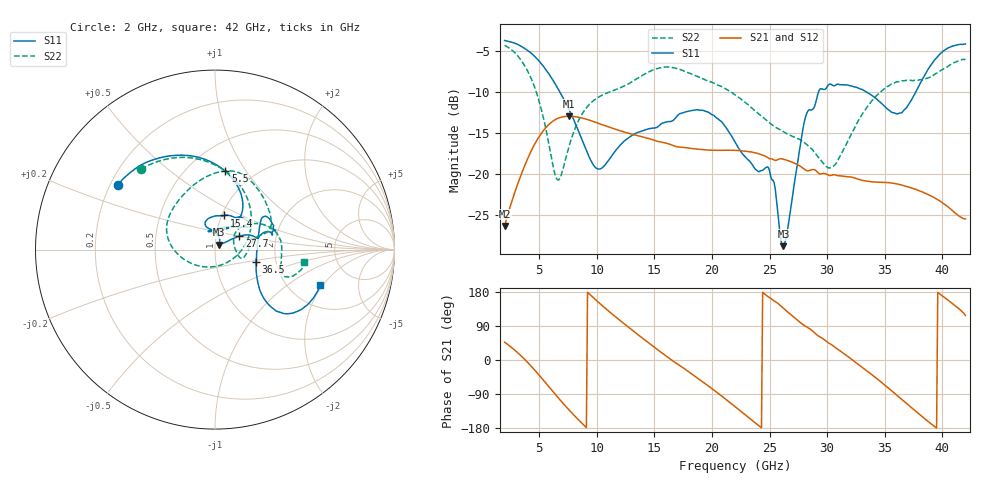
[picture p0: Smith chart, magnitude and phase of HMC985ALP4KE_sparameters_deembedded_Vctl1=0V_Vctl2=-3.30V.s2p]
!s2p File: Measurements: S11, S21, S12, S22
# GHz S dB R 50.0
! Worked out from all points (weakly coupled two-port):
!   401 points, 2 GHz to 42 GHz, reference 50 ohm
!   highest |S21| = -12.95 dB at 7.6 GHz (marker M1); lowest = -26.3 dB at 2 GHz (marker M2)
!   lowest |S11| = -28.8 dB at 26.2 GHz (marker M3), VSWR 1.08, Z = 52.3 + j2.96 ohm
!   |S11| at or under -10 dB: 6.795 GHz to 29.25 GHz (22.46 GHz wide, 125 % of centre); 33.41 GHz to 37.69 GHz (4.286 GHz wide, 12.1 % of centre)
!   |S22| runs from -20.7 to -4.3 dB; largest |S21 - S12| = 0.00059
!   S11 on the Smith chart (normalised r, x): 2 GHz: 0.23, +0.29; 5.5 GHz: 0.75, +0.81; 15.4 GHz: 1.03, +0.41; 27.7 GHz: 1.30, +0.20; 36.5 GHz: 1.57, -0.23; 42 GHz: 2.93, -1.89
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2  -3.73 146.3  -26.31 47.1  -26.30 47.1  -4.32 132.6
3.6  -4.58 119.1  -19.47 5.9  -19.47 5.9  -6.48 90.5
4.6  -5.64 100.2  -16.38 -26.1  -16.37 -26.1  -9.39 58.2
5.5  -7.12 82.5  -14.47 -58.0  -14.47 -58.0  -13.96 20.7
6.6  -9.52 63.8  -13.22 -97.7  -13.22 -97.7  -20.70 -68.8
7.6  -12.17 53.2  -12.95 -132.0  -12.96 -132.0  -16.58 -147.5
8.7  -15.74 54.0  -13.15 -166.6  -13.15 -166.6  -12.73 179.5
10.3  -19.36 90.1  -13.89 148.2  -13.87 148.2  -10.51 154.5
12.6  -15.74 109.2  -14.97 90.2  -14.94 90.2  -9.12 121.4
15.4  -14.11 75.1  -16.05 24.6  -16.06 24.6  -7.08 82.1
19.2  -12.23 33.6  -17.02 -57.5  -17.01 -57.5  -8.39 40.0
22  -16.06 51.7  -17.10 -123.0  -17.12 -123.0  -10.33 18.4
24.9  -19.18 104.2  -18.05 166.5  -18.02 166.5  -13.63 11.0
26.2  -28.77 50.9  -18.18 136.6  -18.21 136.6  -14.84 -3.6
27.7  -16.21 28.8  -19.07 98.1  -19.07 98.1  -15.86 -17.4
28.7  -12.15 12.8  -19.45 77.3  -19.45 77.3  -16.98 -16.9
30.6  -9.25 19.7  -20.07 35.5  -20.08 35.5  -18.95 23.4
33.2  -9.83 34.3  -20.80 -23.1  -20.79 -23.1  -12.40 36.6
35.4  -12.24 11.7  -21.05 -76.3  -21.03 -76.3  -9.21 17.7
36.5  -12.49 -16.6  -21.34 -104.6  -21.35 -104.6  -8.63 7.1
39.5  -5.85 -43.6  -23.03 -179.5  -23.00 -179.4  -7.71 -20.5
42  -4.15 -18.7  -25.44 117.6  -25.42 117.5  -5.98 -7.9
